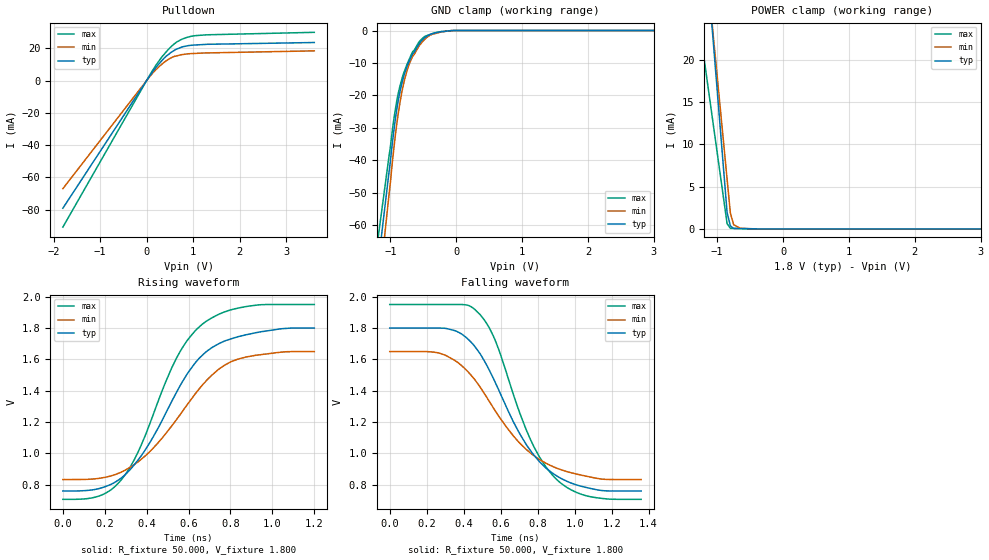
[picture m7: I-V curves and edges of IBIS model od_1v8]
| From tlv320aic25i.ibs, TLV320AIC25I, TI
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[Model]   od_1v8
Model_type I/O_open_drain
Vinl=5.400E-01
Vinh=1.260E+00
Vref=1.800E+00
Rref=5.000E+02
Cref=2.000E-11
Vmeas=9.000E-01
C_comp   1.070E-12   1.070E-12   1.070E-12
[Voltage Range]   1.800E+00   1.650E+00   1.950E+00
[POWER Clamp Reference]   1.800E+00   1.650E+00   1.950E+00
[GND Clamp Reference]   0.000E+00   0.000E+00   0.000E+00
[Pullup Reference]   1.800E+00   1.650E+00   1.950E+00
[Pulldown Reference]   0.000E+00   0.000E+00   0.000E+00
[Temperature Range]   25   85   -40
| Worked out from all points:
|   slope of the pulldown table from 0 to 0.27 V, typ, clamps not added: 25.7 ohm
|   GND clamp passes 1 mA (typ) near -0.36 V on its own axis
|   POWER clamp passes 1 mA (typ) near -0.82 V on its own axis
|   rising waveform, R_fixture 50.000, V_fixture 1.800: 20-80 % time 276ps typ, 298ps min, 245ps max; typ from 0.761 V to 1.8 V
|   falling waveform, R_fixture 50.000, V_fixture 1.800: 20-80 % time 284ps typ, 319ps min, 245ps max; typ from 1.8 V to 0.761 V
[GND Clamp]
-1.8V     -177.3mA   -200.2mA   -157.4mA
-1.02V    -43.67mA   -50.61mA   -38.74mA
-960mV    -33.14mA   -38.86mA   -29.28mA
-900mV    -24.05mA   -28.52mA   -21.48mA
-840mV    -17.65mA   -20.61mA   -16.11mA
-800mV    -14.37mA   -16.57mA   -13.32mA
-740mV    -10.72mA   -11.95mA   -10.13mA
-660mV    -7.159mA   -7.876mA   -6.46mA
-480mV    -2.223mA   -2.767mA   -1.845mA
-360mV    -978.6uA   -1.135mA   -932uA
-40mV     0A         0A         0A
3.6V      0A         0A         0A
[POWER Clamp]
-1.8V     93.46mA    82.75mA    53.72mA
-1V       16.4mA     18.05mA    9.022mA
-850mV    1.946mA    5.92mA     641.4uA
-800mV    370.4uA    1.876mA    73.68uA
-750mV    60.36uA    504.1uA    65.92uA
-650mV    44.27uA    79.79uA    50.41uA
-375mV    0A         0A         7.756uA
3.6V      0A         0A         0A
[Pulldown]
-1.8V     -79.13mA   -67.01mA   -90.85mA
100mV     4.251mA    3.559mA    4.933mA
200mV     8.147mA    6.76mA     9.523mA
380mV     13.97mA    11.37mA    16.37mA
520mV     17.34mA    13.98mA    20.87mA
640mV     19.42mA    15.21mA    23.76mA
760mV     20.79mA    16.04mA    25.62mA
920mV     21.72mA    16.6mA     27.13mA
1.22V     22.28mA    17.04mA    28.16mA
3.6V      23.54mA    18.37mA    29.85mA
[Rising Waveform]
R_fixture = 50.000
V_fixture = 1.800
V_fixture_min = 1.650
V_fixture_max = 1.950
|  time   V(typ)   V(min)   V(max)
0s        760.7mV    833.7mV    707.4mV
170ps     775.1mV    840.7mV    727.3mV
280ps     844.5mV    881.8mV    833.6mV
370ps     977.7mV    958.3mV    1.041V
540ps     1.384V     1.212V     1.602V
600ps     1.52V      1.323V     1.732V
670ps     1.632V     1.443V     1.829V
750ps     1.704V     1.543V     1.891V
850ps     1.749V     1.607V     1.931V
1.2ns     1.8V       1.65V      1.95V
[Falling Waveform]
R_fixture = 50.000
V_fixture = 1.800
V_fixture_min = 1.650
V_fixture_max = 1.950
|  time   V(typ)   V(min)   V(max)
0s        1.8V       1.65V      1.95V
270ps     1.8V       1.639V     1.95V
380ps     1.768V     1.569V     1.95V
460ps     1.683V     1.471V     1.919V
570ps     1.455V     1.273V     1.723V
740ps     1.054V     1.024V     1.146V
810ps     947.7mV    961.3mV    977.5mV
880ps     875.1mV    917.7mV    862.2mV
1.06ns    783.8mV    855.8mV    731mV
1.36ns    760.7mV    833.7mV    707.4mV
[Ramp]
dV/dt_r   6.236E-01/2.761E-10   4.898E-01/2.976E-10   7.456E-01/2.443E-10
dV/dt_f   6.236E-01/2.836E-10   4.898E-01/3.185E-10   7.456E-01/2.438E-10
R_load = 50
